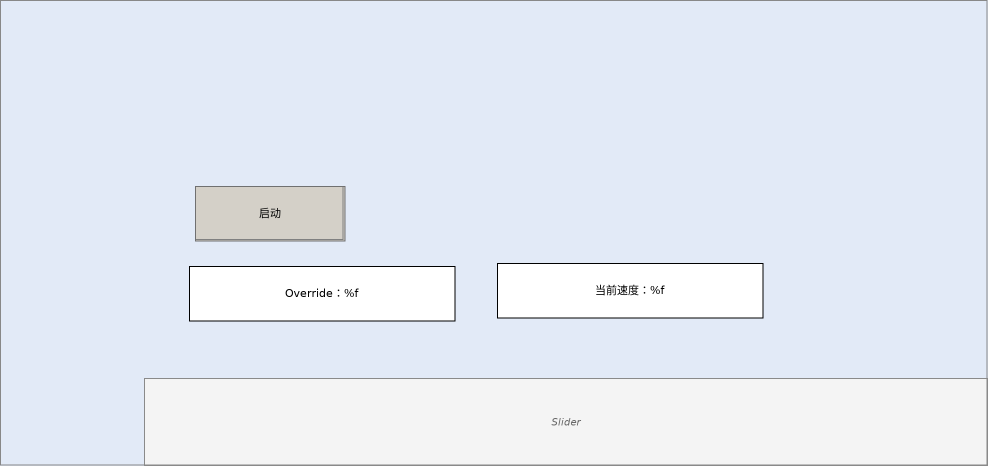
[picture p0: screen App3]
VISUALIZATION App3  // 988x466
    Slider (144,378 844x88), variable: MAIN.lrManualOverride, scale 0..100
    Rectangle (189,266 266x55), "Override：%f", text variable: MAIN.lrManualOverride
    Button (195,186 150x55), "启动"
        toggle MAIN.bStartApp3
    Rectangle (497,263 266x55), "当前速度：%f", text variable: MAIN.Ax1.NcToPlc.ActVelo
END_VISUALIZATION
